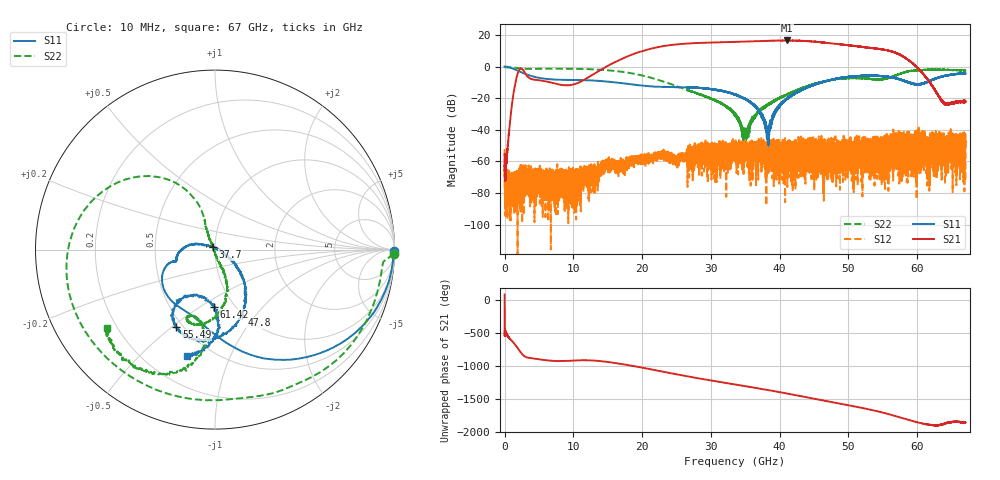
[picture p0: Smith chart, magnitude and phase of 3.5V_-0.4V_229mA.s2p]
! MARKI MICROWAVE INC.
! Date:  10/21/2020
! Model Number:  AMM-7210CH
! Description:  2-port Small Signal S-parameter data for AMM-7210CH
! Frequency Range:  10 MHz to 67 GHz
! Port Configuration:  PORT 1: Input
!  PORT 2: Output
! Bias Condition: Vd = +3.5V, Vg = -0.4V
! AMM-7210CH s2p files are only valid for small signal conditions (below -10 dBm input power)
# Hz S  dB  R 50
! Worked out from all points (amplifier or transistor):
!   20001 points, 10 MHz to 67 GHz, reference 50 ohm
!   highest |S21| = 16.5 dB at 41.01 GHz (marker M1)
!   |S21| within 3 dB of that: 23.98 GHz to 49.82 GHz (25.84 GHz wide, 70 % of centre)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
!   unconditionally stable (mu >= 1): start of sweep to end of sweep
!   at 11.17 GHz: K = 1145.81, MAG = -3.4 dB, |S12| = -69.8 dB
!   at 33.51 GHz: K = 32.77, MAG = 15.7 dB, |S12| = -52.1 dB
!   at 67 GHz: K = 448.18, MAG = -16.8 dB, |S12| = -47.7 dB
!   S11 on the Smith chart (normalised r, x): 10 MHz: open; 37.7 GHz: 0.98, +0.03; 47.8 GHz: 0.99, -0.85; 55.49 GHz: 0.46, -0.52; 61.42 GHz: 0.81, -0.57; 67 GHz: 0.39, -0.70
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1e7  -0.03 -0.4  -55.43 79.7  -52.13 -149.9  -0.03 -1.4
2.237418e9  -3.26 -62.8  -1.64 -61.6  -68.67 15.0  -1.20 -61.9
1.117723e10  -8.57 -132.7  -9.33 162.9  -72.45 161.4  -1.50 -168.6
1.707235e10  -10.55 -159.8  4.89 105.4  -62.37 137.8  -3.37 148.5
1.995627e10  -12.01 -164.2  9.67 52.0  -60.54 126.2  -5.63 129.1
2.234112e10  -12.83 -163.4  12.28 3.9  -56.69 108.4  -8.48 116.5
2.464557e10  -13.01 -164.6  13.79 -42.7  -58.79 98.0  -11.81 109.7
2.766012e10  -13.28 -169.9  14.77 -100.6  -48.37 95.6  -16.55 111.6
3.082205e10  -14.96 179.0  15.21 -157.5  -59.03 34.6  -21.91 116.5
3.3505e10  -17.70 168.0  15.57 155.7  -52.06 19.0  -30.29 123.9
3.770192e10  -34.91 125.6  16.15 81.7  -47.56 -15.7  -25.65 -77.0
4.101458e10  -20.69 -30.8  16.46 19.7  -56.61 -128.3  -18.00 -67.9
4.271278e10  -15.85 -39.9  16.34 -14.0  -55.81 -115.2  -14.62 -69.3
4.467223e10  -12.08 -47.9  15.89 -53.5  -51.52 -174.6  -11.57 -76.6
4.780067e10  -8.13 -67.8  14.42 -115.9  -52.67 -101.2  -8.35 -91.5
5.124395e10  -6.06 -91.3  12.78 174.7  -53.53 156.7  -7.27 -108.8
5.357855e10  -5.82 -105.9  11.56 124.1  -47.75 -141.4  -8.06 -111.3
5.548777e10  -6.35 -116.5  10.36 75.9  -55.20 91.8  -7.71 -101.0
5.583612e10  -6.49 -118.6  10.01 65.9  -48.23 157.7  -7.18 -98.3
5.866309e10  -10.02 -123.6  4.18 -20.7  -55.82 68.6  -3.15 -105.6
6.141973e10  -9.96 -90.9  -7.72 -89.7  -44.52 75.2  -2.07 -123.5
6.7e10  -4.46 -104.8  -22.29 -59.9  -47.68 43.7  -2.54 -144.0
